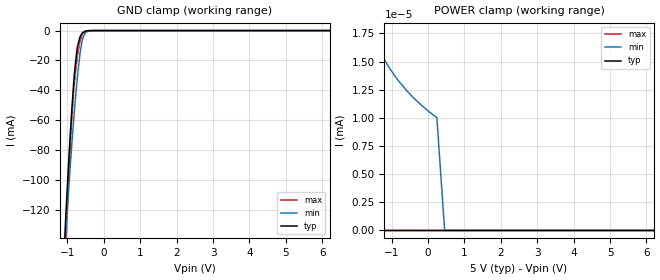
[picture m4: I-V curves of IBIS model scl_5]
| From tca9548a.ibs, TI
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|   scl_5 Model
[Model]   scl_5
Model_type   Input
Vinl = 1.5
Vinh = 3.5
|   typ   min   max
|   (nom PVT)   (fast PVT)   (slow PVT)
C_comp   6.033e-12   5.485e-12   6.668e-12
[Model spec]
|subparameter
Vinl   1.5   1.35   1.65
Vinh   3.5   3.15   3.85
| Where nom  PVT is Nominal Process, 5V, 27C
|   Fast PVT is Strong Process,  5.5V, -40C
|   Slow PVT is Weak Process,   4.5V, 125C
[Voltage Range]   5   4.5   5.5
|Junction Temperature
[Temperature Range]   27   125   -40
[Power Clamp Reference]   5   4.5   5.5
[GND Clamp Reference]   0   0   0
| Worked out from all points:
|   GND clamp passes 1 mA (typ) near -0.55 V on its own axis
[GND Clamp]
|   Voltage   I(typ)   I(min)   I(max)
-5V       -3.271A    -2.584A    -3.951A
-1.14V    -172.5mA   -173.7mA   -206.8mA
-1.046V   -124.9mA   -135.9mA   -146.1mA
-1.035V   -119.9mA   -131.9mA   -139.7mA
-1.013V   -109.5mA   -123.5mA   -126.7mA
-886mV    -55.23mA   -78.29mA   -60.96mA
-803.5mV  -27.54mA   -52.32mA   -33.71mA
-730mV    -11.71mA   -32.19mA   -17.9mA
-645mV    -3.76mA    -13.96mA   -6.374mA
-581mV    -1.387mA   -5.414mA   -2.173mA
-509mV    -368.9uA   -1.285mA   -487.2uA
9.995V    0A         0A         0A
[POWER Clamp]
|   Voltage   I(typ)   I(min)   I(max)
-5V       2.258mA    2.326mA    3.114mA
-1.937V   135.2nA    29.51nA    91.26uA
-1.849V   0A         20.42nA    27.05uA
-1.782V   0A         19.25nA    3.271uA
-1.25V    0A         15.43nA    0A
-1.036V   0A         14.3nA     0A
-896mV    0A         13.65nA    0A
-610mV    0A         12.5nA     0A
-180.5mV  0A         11.12nA    0A
242.5mV   0A         10.01nA    0A
456mV     0A         0A         0A
9.995V    0A         0A         0A
